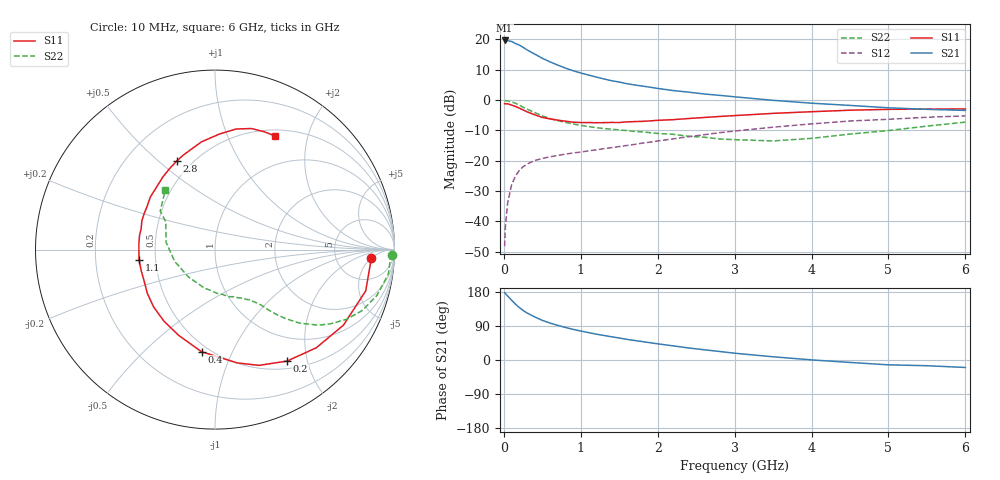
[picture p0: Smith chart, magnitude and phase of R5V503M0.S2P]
! SIEMENS Small Signal Semiconductors
! BFR183
! Si NPN RF Bipolar Junction Transistor in SOT23
! VCE = 0.5 V  IC = 3 mA
! Common Emitter S-Parameters:  May  1996
# GHz  S  MA  R  50
!  f  S11  S21  S12  S22
! GHz  MAG  ANG  MAG  ANG  MAG  ANG  MAG  ANG
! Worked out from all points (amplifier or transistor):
!   36 points, 10 MHz to 6 GHz, reference 50 ohm
!   highest |S21| = 19.7 dB at 10 MHz (marker M1)
!   |S21| within 3 dB of that: start of sweep to 294.9 MHz
!   unconditionally stable (mu >= 1): 1.143 GHz to 3.58 GHz
!   at 250 MHz: K = 0.31, MSG = 19.7 dB, |S12| = -22.0 dB
!   at 1.4 GHz: K = 1.09, MAG = 9.2 dB, |S12| = -15.7 dB
!   at 6 GHz: K = 0.98, MSG = 0.9 dB, |S12| = -5.2 dB
!   S11 on the Smith chart (normalised r, x): 10 MHz: 13, -5; 200 MHz: 0.61, -1.67; 400 MHz: 0.45, -0.77; 1.1 GHz: 0.40, -0.06; 2.8 GHz: 0.41, +0.57; 6 GHz: 0.58, +1.50
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0.01  0.8731 -3.2  9.643 178.1  0.0039 88.6  0.9884 -1.6
0.02  0.8684 -6.1  9.497 175.4  0.0082 85.9  0.9782 -3.3
0.05  0.8707 -15.3  9.537 168.8  0.0203 81.3  0.9753 -8.1
0.1  0.8305 -30.4  9.286 158.0  0.0395 73.7  0.937 -15.9
0.15  0.786 -44.1  8.589 147.6  0.0557 66.4  0.8875 -22.5
0.2  0.7396 -57.1  8.101 138.7  0.0689 61.0  0.8285 -28.0
0.25  0.69 -69.2  7.443 130.7  0.0795 55.6  0.7651 -32.7
0.3  0.6433 -78.9  6.76 124.3  0.088 52.4  0.7131 -36.2
0.4  0.574 -97.5  5.758 113.8  0.1009 47.1  0.6242 -41.0
0.5  0.5194 -112.8  4.907 104.6  0.1089 44.1  0.5489 -44.4
0.6  0.4898 -125.5  4.281 97.5  0.116 42.2  0.4964 -46.6
0.7  0.4681 -136.9  3.786 91.4  0.1225 41.4  0.4596 -48.0
0.9  0.4325 -155.7  3.057 80.9  0.1345 40.9  0.4043 -50.2
1.1  0.4269 -172.3  2.592 72.4  0.1455 41.9  0.3665 -52.9
1.3  0.4255 175.2  2.236 64.8  0.1583 42.5  0.3399 -55.4
1.6  0.4379 158.5  1.865 54.4  0.1785 43.5  0.314 -60.2
2.2  0.4761 133.4  1.439 37.3  0.2293 43.7  0.273 -73.9
2.8  0.5371 113.5  1.2 22.6  0.2896 40.4  0.2289 -95.9
3.5  0.6048 97.2  0.993 8.5  0.3578 33.1  0.2123 -133.9
4.5  0.6819 80.1  0.818 -6.4  0.4526 20.6  0.2755 171.5
5.5  0.7122 67.0  0.705 -15.1  0.5212 8.7  0.3727 144.9
6  0.7155 62.0  0.677 -19.7  0.5502 0.7  0.433 129.8
